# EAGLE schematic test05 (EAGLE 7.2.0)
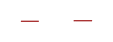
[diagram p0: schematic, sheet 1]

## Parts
R3_3  160 +/- 10%  GENERIC-RESISTOR_  (no package)
Unconnected: R3_3.1 R3_3.2

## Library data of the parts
R3_3 = PickerDesign:GENERIC-RESISTOR_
